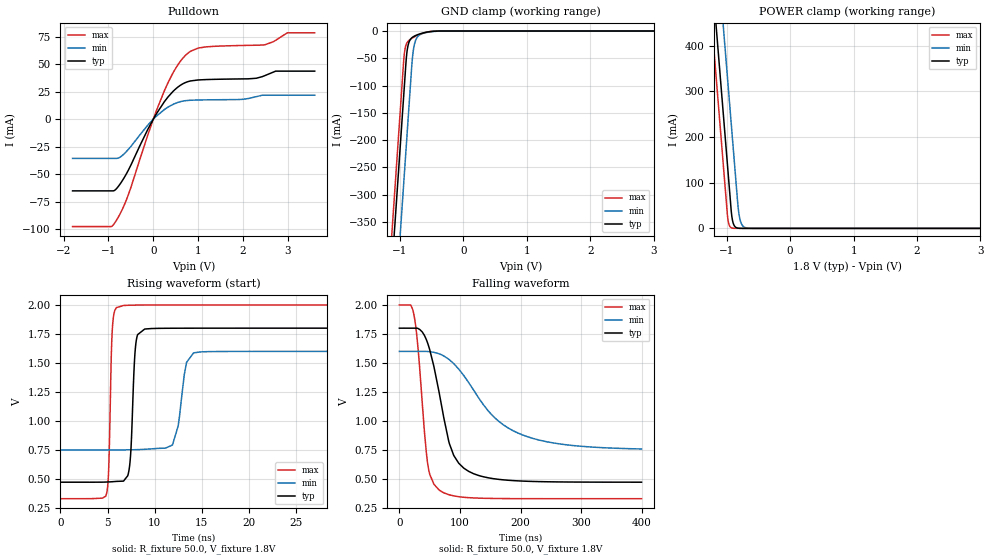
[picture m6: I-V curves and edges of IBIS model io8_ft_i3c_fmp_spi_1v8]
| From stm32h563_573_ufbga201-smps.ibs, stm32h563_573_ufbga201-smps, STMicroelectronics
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[Model]   io8_ft_i3c_fmp_spi_1v8
Model_type I/O_open_drain
Polarity   Non-Inverting
Enable   Active-Low
| CAP_THRESHOLD on pad IOFT is "UDTCAPC" :
| Rising=20.0% of vddiom   Falling=80.0% of vddiom
| C_comp min and max val. don't necessarily correlate with the min and max pvt
| but are the smallest and greatest pad capacitance found.
| var   typ   min   max
C_comp   3.74971pF  3.68797pF  3.87352pF
|C_comp_pulldown   3.74971pF  3.68797pF  3.87352pF
Vinl = 800.0mV
Vinh = 1.0V
Vmeas = 900.0mV   | Reference voltage for timing measurements
Cref  = 50.0pF   | Timing specification test load capacitance value
Rref  = 1.0MOhm   | Timing specification test load resistance value
Vref  = 990.0mV   | Timing specification test load voltage
[Model Spec]
| TIME_THRESHOLD on pin ZII2CV11 is "CMOS" :
| Rising=40.0% of vdd   Falling=60.0% of vdd
Vinl 703.80000mV 631.80000mV 784.80000mV
Vinh 1.06220V 937.20000mV 1.16620V
| variable   typ   min   max
[Temperature Range] 25.0 125.0 -40.0
| variable   typ   min   max
[Voltage Range] 1.8V 1.6V 2.0V
| variable   typ   min   max
[POWER Clamp Reference] 1.8V 1.6V 2.0V
| variable   typ   min   max
[GND Clamp Reference] 0V 0V 0V
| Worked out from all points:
|   slope of the pulldown table from 0 to 0.27 V, typ, clamps not added: 15.8 ohm
|   GND clamp passes 1 mA (typ) near -0.52 V on its own axis
|   POWER clamp passes 1 mA (typ) near -0.84 V on its own axis
|   rising waveform, R_fixture 50.0, V_fixture 1.8V: 20-80 % time 403ps typ, 856ps min, 285ps max; typ from 0.474 V to 1.8 V
|   falling waveform, R_fixture 50.0, V_fixture 1.8V: 20-80 % time 33.3ns typ, 83.6ns min, 15.8ns max; typ from 1.8 V to 0.474 V
[POWER Clamp]
-1.8V     1.518A     1.709A     1.407A
-1.23V    548.8mA    740.2mA    437.5mA
-1.16V    429.8mA    621.2mA    318.5mA
-1.05V    242.8mA    434.2mA    131.5mA
-980mV    123.8mA    315.2mA    17.95mA
-930mV    38.81mA    230.2mA    1.49mA
-910mV    17.82mA    196.2mA    550.8uA
-890mV    8.18mA     162.2mA    203.5uA
-810mV    363.5uA    33.6mA     3.797uA
-770mV    76.62uA    10.47mA    518.8nA
-710mV    7.416uA    1.822mA    26.34nA
3.6V      0A         0A         0A
[GND Clamp]
-1.8V     -1.579A    -1.74A     -1.515A
-1.24V    -627.3mA   -788.3mA   -562.7mA
-1.05V    -304.3mA   -465.3mA   -239.7mA
-940mV    -117.3mA   -278.3mA   -52.69mA
-930mV    -100.3mA   -261.3mA   -40.52mA
-900mV    -50.11mA   -210.3mA   -24.23mA
-880mV    -30.95mA   -176.3mA   -20.02mA
-810mV    -12.18mA   -57.97mA   -13.23mA
-780mV    -9.807mA   -29.1mA    -11.19mA
-690mV    -5.41mA    -7.142mA   -6.184mA
-420mV    -170.4uA   -446.1uA   -81.94uA
3.6V      5.755nA    953.4nA    228.2pA
| variable   typ   min   max
[Pullup Reference] 1.8V 1.6V 2.0V
| variable   typ   min   max
[Pulldown Reference] 0V 0V 0V
[Pulldown]
-1.8V     -65.02mA   -35.56mA   -97.42mA
-940mV    -65.02mA   -35.56mA   -97.42mA
-850mV    -64.17mA   -35.56mA   -93.49mA
-570mV    -47.32mA   -28.01mA   -70.04mA
-120mV    -9.088mA   -5.279mA   -14.07mA
250mV     16.04mA    8.831mA    26.05mA
520mV     28.19mA    14.82mA    47.53mA
780mV     34.17mA    17.07mA    60.14mA
1.18V     35.97mA    17.56mA    65.65mA
2.49V     39.57mA    21.77mA    67.55mA
2.99V     43.62mA    21.77mA    78.38mA
3.6V      43.62mA    21.77mA    78.38mA
[Ramp]
dV/dt_r 795.76119mV/399.7227ps 508.89748mV/790.11147ps 1.00097V/282.78564ps
dV/dt_f 795.72529mV/32.65092ns 504.04593mV/83.28219ns 1.00099V/15.80725ns
R_load = 50.0
| Removed startup time: 0s 0s 0s  .
| Removed end time: 36.4ns.
[Rising Waveform]
R_fixture   = 50.0
V_fixture   = 1.8V
V_fixture_min = 1.6V
V_fixture_max = 2.0V
0s        473.7mV    751.8mV    331.7mV
4.85ns    475mV      751.7mV    362.1mV
5.5ns     477.7mV    751.9mV    1.775V
5.95ns    480.4mV    751.9mV    1.977V
7.25ns    561.9mV    752.3mV    1.997V
8ns       1.659V     753.5mV    1.998V
8.95ns    1.792V     756.7mV    1.999V
11.9ns    1.799V     793.7mV    2V
14.15ns   1.8V       1.587V     2V
36.4ns    1.8V       1.6V       2V
| Removed startup time: 0s 0s 0s  .
| Removed end time: 399.4ns.
[Falling Waveform]
R_fixture   = 50.0
V_fixture   = 1.8V
V_fixture_min = 1.6V
V_fixture_max = 2.0V
0s        1.8V       1.6V       2V
23.5ns    1.8V       1.6V       1.929V
30.6ns    1.798V     1.6V       1.637V
46.45ns   1.674V     1.599V     642.6mV
65.2ns    1.257V     1.58V      408.2mV
89.65ns   704.6mV    1.495V     356mV
122.3ns   547.1mV    1.268V     338.3mV
163.1ns   498.6mV    1.002V     333.2mV
211.9ns   481.5mV    864.2mV    331.9mV
399.4ns   473.8mV    759.9mV    331.7mV
